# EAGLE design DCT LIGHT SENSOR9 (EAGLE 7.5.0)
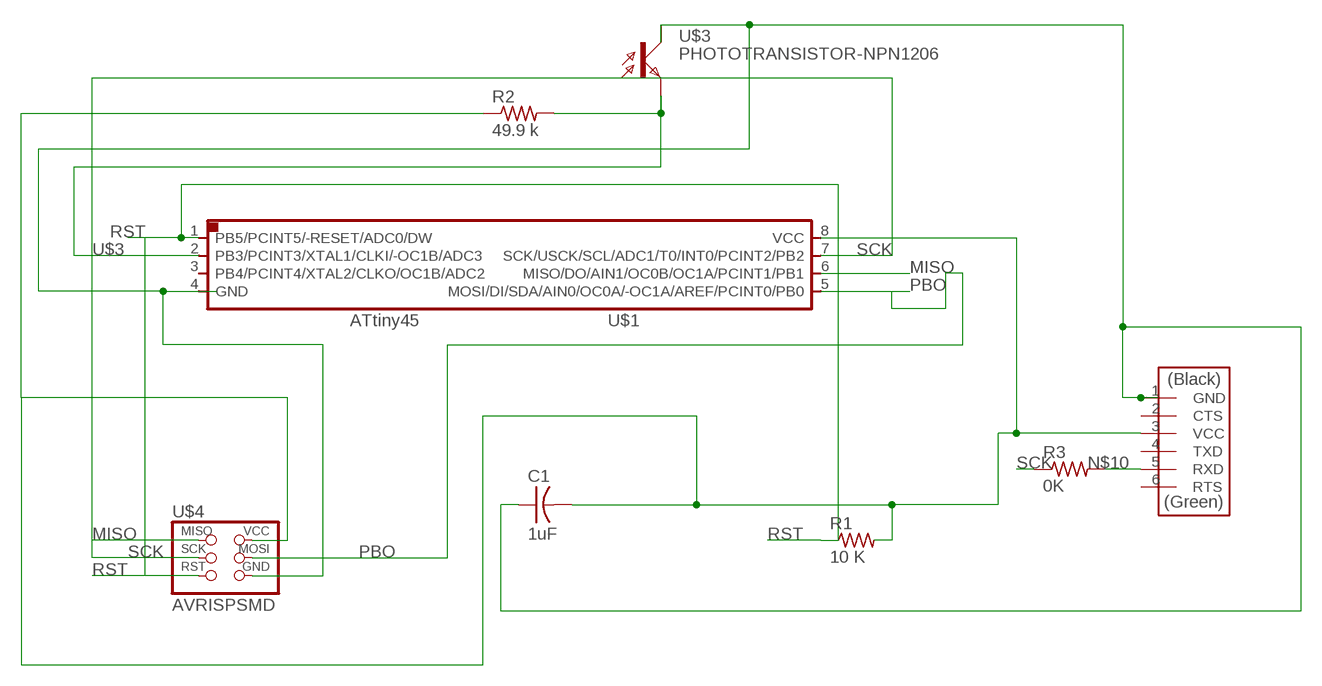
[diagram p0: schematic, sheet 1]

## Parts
C1  1uF  CAP-US1206FAB  [C1206FAB]
R1  10 K  RES-US1206FAB  [R1206FAB]
R2  49.9 k  RES-US1206FAB  [R1206FAB]
R3  0K  RES-US1206FAB  [R1206FAB]
U$1  ATTINY45SI  [SOIC8]
U$2  FTDI-SMD-HEADER  [1X06SMD]
U$3  PHOTOTRANSISTOR-NPN1206  [OP1206]
U$4  AVRISPSMD  [2X03SMD]

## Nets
MISO: U$1.6(MISO/DO/AIN1/OC0B/OC1A/PCINT1/PB1) U$4.1(MISO)
N$2: C1.1 U$2.1(GND) U$3.COLLECTOR(C) U$4.6(GND)
N$9: C1.2 R1.2 R2.1 U$1.8(VCC) U$2.3(VCC) U$4.2(VCC)
N$10: R3.2 U$2.5(RXD)
PBO: U$1.5(MOSI/DI/SDA/AIN0/OC0A/-OC1A/AREF/PCINT0/PB0) U$4.4(MOSI)
RST: R1.1 U$1.1(PB5/PCINT5/-RESET/ADC0/DW) U$4.5(RST)
SCK: R3.1 U$1.7(SCK/USCK/SCL/ADC1/T0/INT0/PCINT2/PB2) U$4.3(SCK)
U$3: R2.2 U$1.2(PB3/PCINT3/XTAL1/CLKI/-OC1B/ADC3) U$3.EMITTER(E)
Unconnected: U$1.3(PB4/PCINT4/XTAL2/CLKO/OC1B/ADC2) U$1.4(GND) U$2.2(CTS) U$2.4(TXD) U$2.6(RTS)

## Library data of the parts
C1 = fab:CAP-US
R1-R3 = fab:RES-US: Resistor (US Symbol)
U$1 = fab:ATTINY45
U$2 = fab:FTDI-SMD-HEADER
U$3 = fab:PHOTOTRANSISTOR-NPN
U$4 = fab:AVRISP

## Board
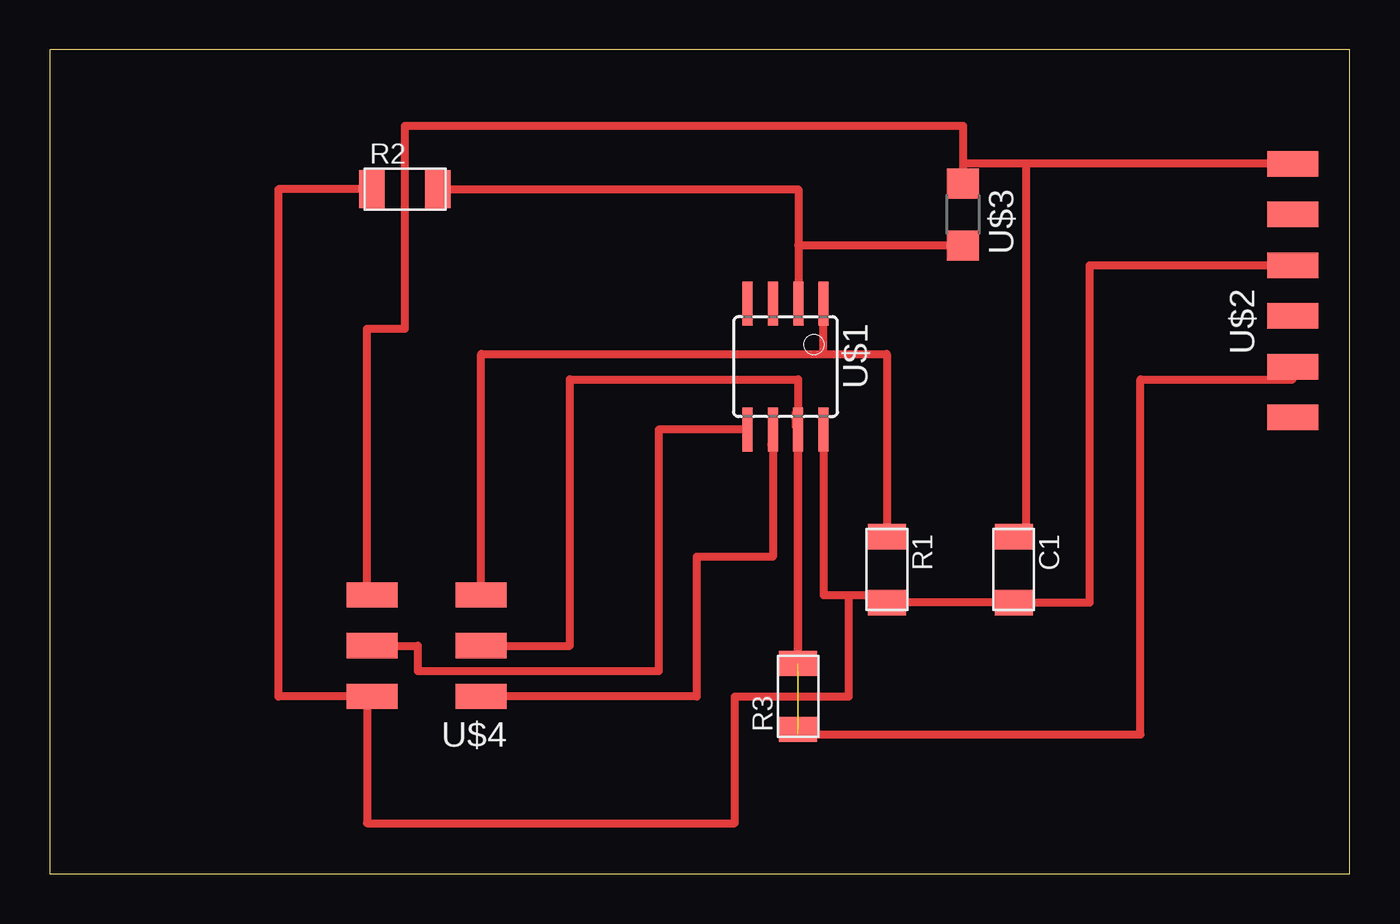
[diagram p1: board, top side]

Size 65.08 x 41.27 mm. Coordinates in mm from the lower left corner, seen from the top.
Outline: 0,0 65.08,0 65.08,41.27 0,41.27 0,0
Copper layers (1*16): Top 0.035mm / dielectric 1.5mm / Bottom 0.035mm
Design rules "default": minimum track width 10mil, minimum drill 24mil, track to track 8mil, track to pad 8mil, pad to pad 8mil, via to via 8mil, smd to smd 8mil, copper to edge 40mil, drill to drill 8mil, minimum pad ring 10mil, minimum via ring 8mil, stop-mask expansion 4mil, vias tented up to drill 0mil, thermal gap 10mil

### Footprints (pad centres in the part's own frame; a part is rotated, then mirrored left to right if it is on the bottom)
C1206FAB = smd 1.27 x 1.905: 1 -1.651,0; 2 1.651,0
R1206FAB = smd 1.27 x 1.905: 1 -1.651,0; 2 1.651,0
SOIC8 = smd 0.5 x 2.2: 1 -1.905,-3.154; 2 -0.645,-3.154; 3 0.625,-3.154; 4 1.895,-3.154; 5 1.905,3.154; 6 0.635,3.154; 7 -0.635,3.154; 8 -1.905,3.154
1X06SMD = smd 2.54 x 1.27: 1 0,6.35; 2 0,3.81; 3 0,1.27; 4 0,-1.27; 5 0,-3.81; 6 0,-6.35
OP1206 = smd 1.5 x 1.6: COLLECTOR -1.55,0; EMITTER 1.55,0
2X03SMD = smd 2.54 x 1.27: 1 -2.54,2.54; 2 2.92,2.54; 3 -2.54,0; 4 2.92,0; 5 -2.54,-2.54; 6 2.92,-2.54

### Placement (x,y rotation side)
C1  48.26,15.24 270 top
R1  41.91,15.24 270 top
R2  17.78,34.29 0 top
R3  37.47,8.89 90 top
U$1  36.83,25.4 180 top
U$2  62.23,29.21 0 top
U$3  45.72,33.02 270 top
U$4  19.05,11.43 180 top

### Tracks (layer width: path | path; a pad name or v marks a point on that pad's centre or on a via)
MISO
  Top 0.254: 36.12,21.49 36.12,22.17 U$1.6 | 23.55,8.91 21.72,8.91 U$4.1
  Top 0.406: 36.12,21.49 36.2,21.49 36.2,15.88 32.38,15.88 32.38,8.89 U$4.1
N$2
  Top 0.406: U$2.1 48.9,35.56 | 48.9,35.56 45.72,35.56 U$3.COLLECTOR 45.72,37.47 17.78,37.47 17.78,27.3 15.88,27.3 15.88,13.97 U$4.6 | C1.1 48.9,16.89 48.9,35.56
N$9
  Top 0.406: U$2.3 52.07,30.48 52.07,13.59 C1.2 R1.2 41.91,13.97 40.01,13.97 | U$4.2 11.43,8.89 11.43,34.29 R2.1 | U$1.8 38.73,13.97 40.01,13.97 | U$4.2 16.51,8.89 | U$4.2 15.88,8.89 15.88,2.54 34.29,2.54 34.29,8.89 40.01,8.89 40.01,13.97
N$10  (1 unrouted)
  Top 0.406: 37.47,6.99 54.61,6.99 54.61,24.77 62.23,24.77 U$2.5 | R3.2 37.47,22.23
PBO
  Top 0.406: U$1.5 30.48,22.25 30.48,10.16 18.41,10.16 18.41,11.43 U$4.4
RST
  Top 0.406: U$4.5 21.59,26.04 38.73,26.04 | 38.73,26.04 U$1.1 | 38.73,26.04 41.91,26.04 R1.1
SCK  (1 unrouted)
  Top 0.254: 37.26,23.09 37.26,22.4 U$1.7 | 21.72,11.43 U$4.3
  Top 0.406: 21.72,11.43 26.04,11.43 26.04,24.77 37.47,24.77 U$1.7 37.47,10.16
U$3
  Top 0.406: R2.2 37.48,34.29 37.48,31.47 | 37.48,31.47 U$1.2 | U$3.EMITTER 37.48,31.47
